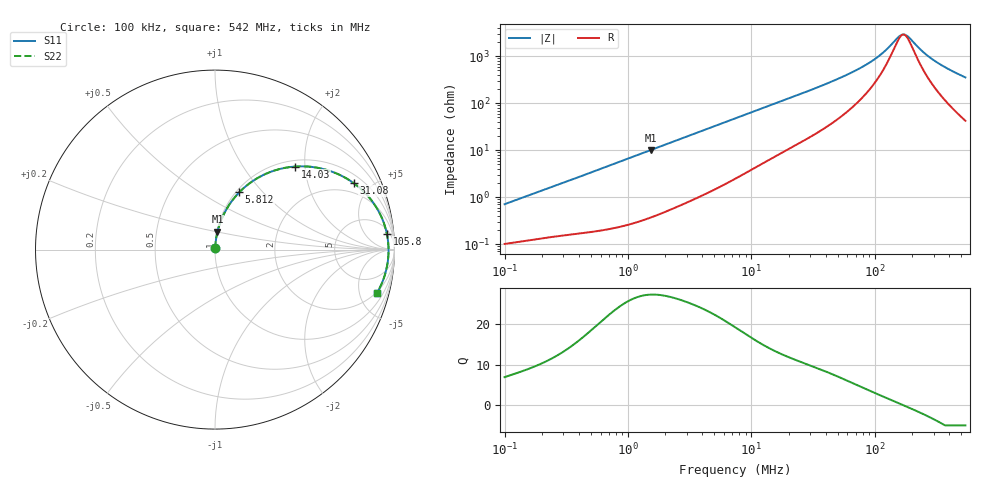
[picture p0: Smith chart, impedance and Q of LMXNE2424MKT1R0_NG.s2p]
! LMXNE2424MKT1R0_NG  S-PARAMETER MODEL  ( General Type )
! Model Generated by TAIYO YUDEN Corporation (http://www.ty-top.com)
! Version 1.0
! TAIYO YUDEN Control No. 191023NI43SB-FBB
! Copyright(c) 2019 TAIYO YUDEN CO.,LTD. All Rights Reserved.
! Product Description (link to TY-COMPAS)
! https://ds.yuden.co.jp/TYCOMPAS/or/detail?pn=LMXNE2424MKT1R0NNG&u=M
! Products Name : Inductors
! Characteristics :
!  Inductance : 1.0 uH , SRF(min) : 101 MHz , DC Resistance(max) : 0.0924 Ohm
!  Rated Current : Saturation :2350 mA , Temp Rise : 1300 mA
!  Case Size : 2.4 x 2.4 / 0.094 x 0.094 [mm/inch] , Thickness : 1.2 / 0.047 [mm/inch]
!  (Conditions: Temperature = 25 degC , DC Bias Current/Voltage = 0A / 0V)
! External Node Assignments :
!  1  o---GGG---o  2
! GND o---------o GND
! Frequency Range : 0.1MHz  -  542.002916MHz  [ 402 STEP ]
# MHz S RI R 50
! Freq[MHz].  S11 Real  S11 Imag  S21 Real  S21 Imag  S12 Real  S12 Imag  S22 Real  S22 Imag
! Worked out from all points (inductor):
!   401 points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, 100 kHz to 542 MHz, reference 50 ohm
!   read as one part in series: L = 1.11 uH near 104.4 kHz
!   highest Q = 27.4 at 1.533 MHz (marker M1), where L = 1.05 uH
!   self-resonance near 170.5 MHz
!   S11 on the Smith chart (normalised r, x): 100 kHz: 1.00, +0.01; 5.812 MHz: 1.04, +0.75; 14.03 MHz: 1.13, +1.78; 31.08 MHz: 1.41, +3.91; 105.8 MHz: 8, +18; 542 MHz: 1.85, -7.06
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0.1  0.00106 0.00701  0.9989 -0.00701  0.9989 -0.00701  0.00106 0.00701
0.422129  0.0025 0.0282  0.9975 -0.0282  0.9975 -0.0282  0.0025 0.0282
1.533012  0.0137 0.0994  0.9863 -0.0994  0.9863 -0.0994  0.0137 0.0994
1.78193  0.0177 0.1148  0.9823 -0.1148  0.9823 -0.1148  0.0177 0.1148
3.46957  0.0564 0.2114  0.9436 -0.2114  0.9436 -0.2114  0.0564 0.2114
5.811868  0.135 0.319  0.865 -0.319  0.865 -0.319  0.135 0.319
7.362085  0.1956 0.3716  0.8044 -0.3716  0.8044 -0.3716  0.1956 0.3716
14.02978  0.4464 0.4629  0.5536 -0.4629  0.5536 -0.4629  0.4464 0.4629
20.21836  0.6104 0.4472  0.3896 -0.4472  0.3896 -0.4472  0.6104 0.4472
31.0775  0.7719 0.371  0.2281 -0.371  0.2281 -0.371  0.7719 0.371
43.8335  0.861 0.2881  0.139 -0.2881  0.139 -0.2881  0.861 0.2881
63.1686  0.919 0.1994  0.081 -0.1994  0.081 -0.1994  0.919 0.1994
83.53265  0.9445 0.1372  0.0555 -0.1372  0.0555 -0.1372  0.9445 0.1372
105.8136  0.9574 0.0891  0.0426 -0.0891  0.0426 -0.0891  0.9574 0.0891
131.1872  0.964 0.0481  0.036 -0.0481  0.036 -0.0481  0.964 0.0481
159.1866  0.9666 0.0125  0.0334 -0.0125  0.0334 -0.0125  0.9666 0.0125
177.248  0.9669 -0.00707  0.0331 0.00707  0.0331 0.00707  0.9669 -0.00707
189.0542  0.9667 -0.0188  0.0333 0.0188  0.0333 0.0188  0.9667 -0.0188
244.6845  0.9627 -0.067  0.0373 0.067  0.0373 0.067  0.9627 -0.067
296.9077  0.9559 -0.1052  0.0441 0.1052  0.0441 0.1052  0.9559 -0.1052
392.6237  0.9384 -0.1654  0.0616 0.1654  0.0616 0.1654  0.9384 -0.1654
542.0029  0.9018 -0.2436  0.0982 0.2436  0.0982 0.2436  0.9018 -0.2436
